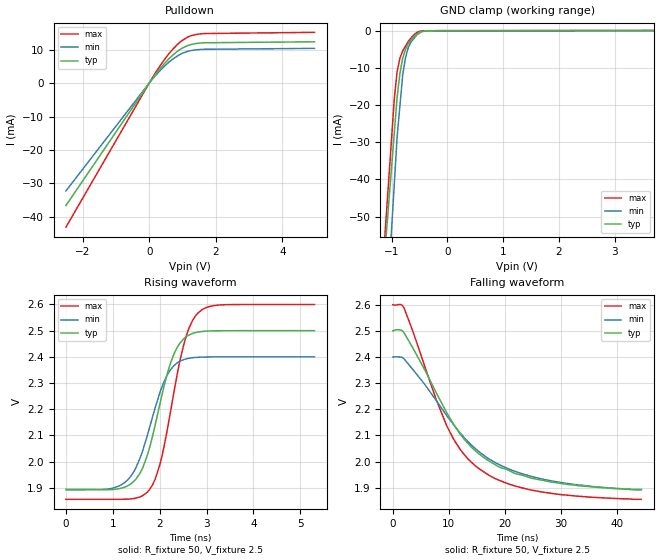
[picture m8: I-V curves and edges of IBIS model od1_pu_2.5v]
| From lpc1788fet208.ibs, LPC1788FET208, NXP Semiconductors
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[Model]   od1_pu_2.5v
Model_type I/O_open_drain
Vinl=7.500E-01
Vinh=1.750E+00
Vref=2.500E+00
Rref=2.000E+03
Cref=0.000E+00
Vmeas=1.250E+00
C_comp   1.240E-12   1.180E-12   1.300E-12
[Voltage Range]   2.500E+00   2.400E+00   2.600E+00
[POWER Clamp Reference]   2.500E+00   2.400E+00   2.600E+00
[GND Clamp Reference]   0.000E+00   0.000E+00   0.000E+00
[Pullup Reference]   2.500E+00   2.400E+00   2.600E+00
[Pulldown Reference]   0.000E+00   0.000E+00   0.000E+00
[Temperature Range]   25   85   -40
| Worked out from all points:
|   slope of the pulldown table from 0 to 0.375 V, typ, clamps not added: 76.6 ohm
|   GND clamp passes 1 mA (typ) near -0.55 V on its own axis
|   rising waveform, R_fixture 50, V_fixture 2.5: 20-80 % time 518ps typ, 542ps min, 493ps max; typ from 1.89 V to 2.5 V
|   falling waveform, R_fixture 50, V_fixture 2.5: 20-80 % time 11.3ns typ, 12.9ns min, 9.37ns max; typ from 2.5 V to 1.89 V
[GND Clamp]
-2.5V     -320.9mA   -428.2mA   -355.8mA
-950mV    -27.31mA   -41.03mA   -18.18mA
-900mV    -17.84mA   -28.54mA   -11.01mA
-850mV    -11.49mA   -20.22mA   -7.415mA
-800mV    -7.413mA   -11.9mA    -5.476mA
-750mV    -5.014mA   -7.253mA   -4.181mA
-700mV    -3.535mA   -4.543mA   -2.887mA
-650mV    -2.594mA   -3.07mA    -2.015mA
-550mV    -1.057mA   -1.212mA   -539.5uA
-400mV    -147.5uA   -112.4uA   -63.11uA
-200mV    -36.9uA    -30.37uA   -38.72uA
5V        16.89uA    16.03uA    16.38uA
[Pulldown]
-2.5V     -36.61mA   -32.23mA   -43.08mA
172.9mV   2.386mA    2.077mA    2.845mA
611.7mV   7.486mA    6.438mA    9.04mA
930.8mV   10.09mA    8.595mA    12.29mA
1.25V     11.52mA    9.708mA    14.13mA
1.609V    12.03mA    10.08mA    14.78mA
4.96V     12.34mA    10.38mA    15.17mA
[Rising Waveform]
R_fixture = 50
V_fixture = 2.5
V_fixture_min = 2.4
V_fixture_max = 2.6
0s        1.894V     1.893V     1.856V
1.25ns    1.902V     1.92V      1.856V
1.585ns   1.957V     2.015V     1.865V
1.783ns   2.053V     2.13V      1.893V
2.031ns   2.242V     2.277V     2.008V
2.3ns     2.409V     2.366V     2.262V
2.576ns   2.478V     2.393V     2.486V
2.7ns     2.489V     2.397V     2.539V
2.9ns     2.497V     2.399V     2.58V
5.301ns   2.5V       2.4V       2.6V
[Falling Waveform]
R_fixture = 50
V_fixture = 2.5
V_fixture_min = 2.4
V_fixture_max = 2.6
0s        2.5V       2.4V       2.6V
1.948ns   2.494V     2.394V     2.59V
7.691ns   2.266V     2.236V     2.24V
9.589ns   2.189V     2.177V     2.139V
12.04ns   2.105V     2.11V      2.047V
15.03ns   2.036V     2.044V     1.979V
18.93ns   1.98V      1.99V      1.929V
24.72ns   1.937V     1.944V     1.891V
32.45ns   1.91V      1.913V     1.869V
44.4ns    1.894V     1.893V     1.856V
[Ramp]
dV/dt_r   3.6354E-01/5.1510E-10   3.0443E-01/5.3810E-10   4.4652E-01/4.9250E-10
dV/dt_f   3.6354E-01/1.1265E-08   3.0443E-01/1.2924E-08   4.4652E-01/9.3583E-09
R_load = 50
